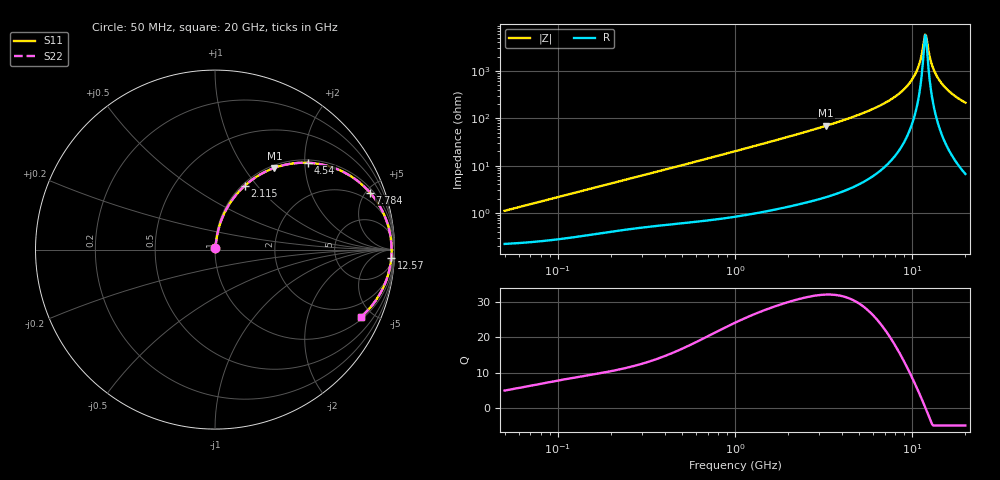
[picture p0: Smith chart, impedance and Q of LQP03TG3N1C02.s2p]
!Murata Part Number: LQP03TG3N1C02
!These Parameters are Measured in Series Mode Connection
!  o--[Z]--o
!Port1  Port2
!  o-------o
!Freq. Start=50[MHz] Stop=20[GHz], 401[Steps]
# Hz S RI R 50
!Freq.(Hz) S11(Real) S11(Imag) S21(Real) S21(Imag) S12(Real) S12(Imag) S22(Real) S22(Imag)
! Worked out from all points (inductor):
!   401 points, 50 MHz to 20 GHz, reference 50 ohm
!   read as one part in series: L = 3.46 nH near 51.52 MHz
!   highest Q = 32.2 at 3.265 GHz (marker M1), where L = 3.39 nH
!   self-resonance near 11.84 GHz
!   S11 on the Smith chart (normalised r, x): 50 MHz: 1.00, +0.02; 2.115 GHz: 1.03, +0.86; 4.54 GHz: 1.07, +2.08; 7.784 GHz: 1.28, +5.31; 12.57 GHz: 14, -38; 20 GHz: 1.13, -4.28
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5e7  0.00233 0.0109  0.9977 -0.0109  0.9977 -0.0109  0.00233 0.0109
1.364002e8  0.00408 0.0289  0.9959 -0.0289  0.9959 -0.0289  0.00408 0.0289
3.721004e8  0.011 0.0749  0.989 -0.0749  0.989 -0.0749  0.011 0.0749
1e9  0.0463 0.1904  0.9537 -0.1904  0.9537 -0.1904  0.0463 0.1904
2.114743e9  0.1653 0.3554  0.8347 -0.3554  0.8347 -0.3554  0.1653 0.3554
2.728004e9  0.2505 0.4179  0.7495 -0.4179  0.7495 -0.4179  0.2505 0.4179
3.265178e9  0.3305 0.4551  0.6695 -0.4551  0.6695 -0.4551  0.3305 0.4551
4.539627e9  0.5201 0.4837  0.4799 -0.4837  0.4799 -0.4837  0.5201 0.4837
5.856089e9  0.6896 0.4444  0.3104 -0.4444  0.3104 -0.4444  0.6896 0.4444
7.442007e9  0.8392 0.3436  0.1608 -0.3436  0.1608 -0.3436  0.8392 0.3436
7.784049e9  0.8635 0.3178  0.1365 -0.3178  0.1365 -0.3178  0.8635 0.3178
9.041845e9  0.9308 0.2183  0.0692 -0.2183  0.0692 -0.2183  0.9308 0.2183
1.019291e10  0.9663 0.1269  0.0337 -0.1269  0.0337 -0.1269  0.9663 0.1269
1.098561e10  0.979 0.0662  0.021 -0.0662  0.021 -0.0662  0.979 0.0662
1.166392e10  0.9835 0.0167  0.0165 -0.0167  0.0165 -0.0167  0.9835 0.0167
1.183995e10  0.9839 0.00422  0.0161 -0.00422  0.0161 -0.00422  0.9839 0.00422
1.220001e10  0.9836 -0.0207  0.0164 0.0207  0.0164 0.0207  0.9836 -0.0207
1.257102e10  0.9821 -0.0456  0.0179 0.0456  0.0179 0.0456  0.9821 -0.0456
1.334722e10  0.9753 -0.0949  0.0247 0.0949  0.0247 0.0949  0.9753 -0.0949
1.460232e10  0.9558 -0.1667  0.0442 0.1667  0.0442 0.1667  0.9558 -0.1667
1.670968e10  0.9074 -0.2659  0.0926 0.2659  0.0926 0.2659  0.9074 -0.2659
2e10  0.8136 -0.3742  0.1864 0.3742  0.1864 0.3742  0.8136 -0.3742
